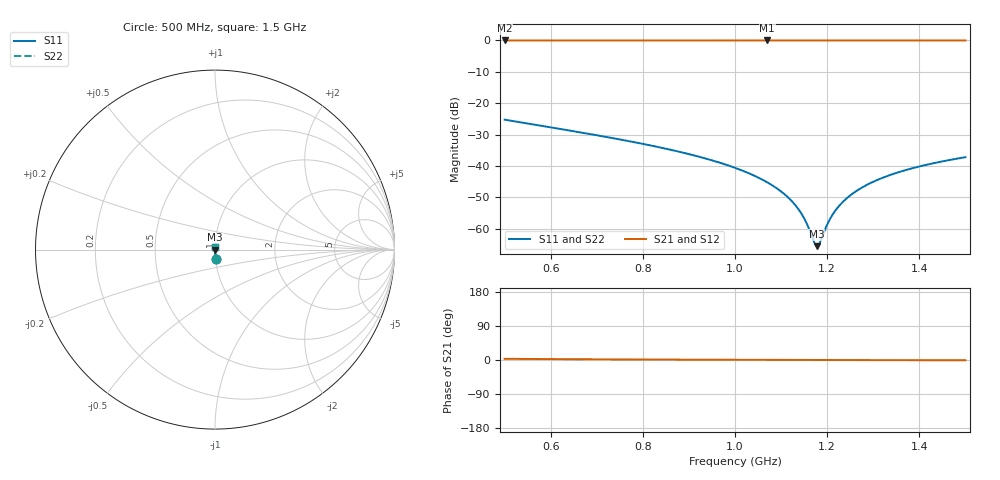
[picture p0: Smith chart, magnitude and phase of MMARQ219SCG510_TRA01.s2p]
! MMARQ219SCG510_TRA01  S-PARAMETER MODEL  ( General Type )
! Model Generated by TAIYO YUDEN Corporation (http://www.ty-top.com)
! Version 1.0
! TAIYO YUDEN Control No. 180601
! Copyright(c) 2018 TAIYO YUDEN CO.,LTD. All Rights Reserved.
! Product Description (link to TY-COMPAS)
! https://ds.yuden.co.jp/TYCOMPAS/or/detail?pn=MMARQ219SCG510JTRA01&u=M
! Products Name : Multilayer Ceramic Capacitors
! Characteristics :
!  Capacitance : 51 pF , Rated Voltage : 250V , TCC : CG / C0G
!  Case Size : 2.0 x 1.25 / 0.079 x 0.049 [mm/inch] , Thickness : 0.85 / 0.033 [mm/inch]
!  (Conditions: Temperature = 25 degC , DC Bias Current/Voltage = 0A / 0V)
! External Node Assignments :
!  1  o---| |---o  2
! GND o---------o GND
! Frequency Range : 500MHz  -  1500MHz  [ 401 STEP ]
# MHz S RI R 50
! Freq[MHz].  S11 Real  S11 Imag  S21 Real  S21 Imag  S12 Real  S12 Imag  S22 Real  S22 Imag
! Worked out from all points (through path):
!   401 points, 500 MHz to 1.5 GHz, reference 50 ohm
!   highest |S21| = 0.00 dB at 1.07 GHz (marker M1); lowest = 0.0 dB at 500 MHz (marker M2)
!   lowest |S11| = -65.6 dB at 1.177 GHz (marker M3), VSWR 1.00, Z = 50.1 - j0.00355 ohm
!   |S11| at or under -10 dB: start of sweep to end of sweep
!   |S22| runs from -65.6 to -25.2 dB; largest |S21 - S12| = 0
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500  0.00336 -0.0546  0.9966 0.0546  0.9966 0.0546  0.00336 -0.0546
667.5  0.00155 -0.0339  0.9985 0.0339  0.9985 0.0339  0.00155 -0.0339
835  0.000828 -0.0199  0.9992 0.0199  0.9992 0.0199  0.000828 -0.0199
927.5  0.000642 -0.0137  0.9994 0.0137  0.9994 0.0137  0.000642 -0.0137
1000  0.000562 -0.00933  0.9994 0.00933  0.9994 0.00933  0.000562 -0.00933
1070  0.000524 -0.00546  0.9995 0.00546  0.9995 0.00546  0.000524 -0.00546
1105  0.000518 -0.00364  0.9995 0.00364  0.9995 0.00364  0.000518 -0.00364
1130  0.000518 -0.00237  0.9995 0.00237  0.9995 0.00237  0.000518 -0.00237
1150  0.00052 -0.00137  0.9995 0.00137  0.9995 0.00137  0.00052 -0.00137
1167.5  0.000523 -0.000518  0.9995 0.000518  0.9995 0.000518  0.000523 -0.000518
1172.5  0.000525 -0.000276  0.9995 0.000276  0.9995 0.000276  0.000525 -0.000276
1177.5  0.000526 -3.54e-05  0.9995 3.54e-05  0.9995 3.54e-05  0.000526 -3.54e-05
1180  0.000527 8.46e-05  0.9995 -8.46e-05  0.9995 -8.46e-05  0.000527 8.46e-05
1185  0.000529 0.000324  0.9995 -0.000324  0.9995 -0.000324  0.000529 0.000324
1200  0.000534 0.00104  0.9995 -0.00104  0.9995 -0.00104  0.000534 0.00104
1210  0.000538 0.00151  0.9995 -0.00151  0.9995 -0.00151  0.000538 0.00151
1222.5  0.000544 0.00209  0.9995 -0.00209  0.9995 -0.00209  0.000544 0.00209
1237.5  0.000552 0.00278  0.9994 -0.00278  0.9994 -0.00278  0.000552 0.00278
1277.5  0.000578 0.00458  0.9994 -0.00458  0.9994 -0.00458  0.000578 0.00458
1335  0.000626 0.00708  0.9994 -0.00708  0.9994 -0.00708  0.000626 0.00708
1410  0.000704 0.0102  0.9993 -0.0102  0.9993 -0.0102  0.000704 0.0102
1500  0.00082 0.0138  0.9992 -0.0138  0.9992 -0.0138  0.00082 0.0138
